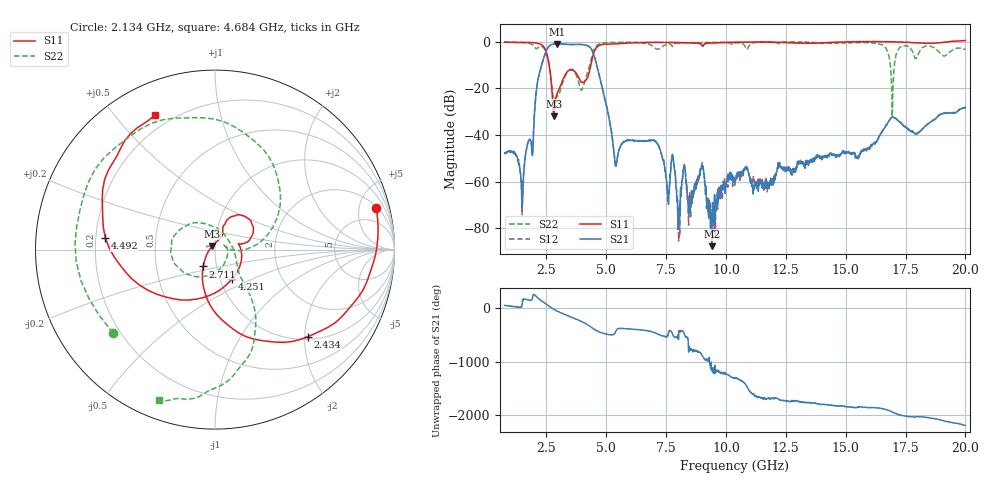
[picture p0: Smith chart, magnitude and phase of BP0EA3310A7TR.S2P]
! s2p File.  Ports: 1,3
# MHz S DB R 50
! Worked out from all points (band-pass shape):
!   1601 points, 750 MHz to 20 GHz, reference 50 ohm
!   highest |S21| = -0.91 dB at 2.94 GHz (marker M1); lowest = -87.8 dB at 9.4 GHz (marker M2)
!   |S21| within 3 dB of the highest: 2.491 GHz to 4.416 GHz (1.925 GHz wide, 55.7 % of centre)
!   lowest |S11| = -32.1 dB at 2.807 GHz (marker M3), VSWR 1.05, Z = 48.4 + j1.9 ohm
!   |S11| at or under -10 dB: 2.611 GHz to 4.348 GHz (1.737 GHz wide, 49.9 % of centre)
!   |S22| runs from -32.2 to 0.0 dB; largest |S21 - S12| = 0.0074
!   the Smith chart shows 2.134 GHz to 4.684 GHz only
!   S11 on the Smith chart (normalised r, x): 2.134 GHz: 2.21, +7.28; 2.434 GHz: 1.07, -2.08; 2.711 GHz: 0.86, -0.16; 4.251 GHz: 1.13, -0.39; 4.492 GHz: 0.24, +0.05; 4.684 GHz: 0.14, +0.64
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750  -0.15 135.7  -47.79 56.6  -47.82 56.8  -0.19 159.8
1495.94  -0.34 80.9  -67.99 133.8  -69.20 122.0  -0.33 118.8
1941.09  -0.41 38.2  -42.93 -107.4  -43.19 -106.6  -1.53 22.8
2133.59  -0.65 14.4  -16.87 -160.7  -16.87 -161.1  -2.69 -140.7
2434.38  -2.98 -43.0  -5.44 99.8  -5.46 99.4  -3.44 76.7
2711.09  -18.85 -124.8  -1.17 9.1  -1.19 8.6  -17.85 -2.7
2807.34  -32.09 128.2  -0.97 -16.9  -1.01 -17.2  -24.74 18.0
2939.69  -22.29 63.4  -0.91 -47.9  -0.94 -48.1  -23.60 13.5
3962.34  -17.45 13.3  -1.14 116.5  -1.16 116.3  -20.80 33.6
4251.09  -14.41 -60.7  -1.86 47.1  -1.85 46.9  -11.96 -49.8
4491.72  -4.24 174.1  -5.97 -28.9  -6.03 -29.3  -3.34 -79.2
4684.22  -1.71 114.2  -13.58 -76.3  -13.55 -76.8  -0.95 -110.5
5394.06  -0.89 7.1  -53.36 -67.6  -53.95 -68.5  -0.27 -165.8
6621.25  -0.36 -75.5  -42.67 -49.0  -42.51 -51.2  -0.60 152.4
7174.69  -0.23 -91.1  -44.53 -123.3  -44.43 -121.3  -3.14 11.9
7583.75  -0.26 -101.3  -66.90 -113.6  -69.11 -108.8  -1.06 -92.9
9003.44  -1.65 -173.7  -52.96 -157.5  -51.83 -153.3  -0.41 -169.1
9400.47  -0.58 168.3  -87.77 -22.3  -72.18 -50.5  -0.24 172.3
10375  -0.14 136.3  -60.22 138.7  -61.30 149.4  -0.60 147.1
13587.34  -0.63 61.0  -51.48 36.2  -51.59 32.5  -0.25 148.9
16799.69  -0.04 22.1  -34.18 -105.6  -34.20 -105.9  -5.95 23.9
20000  0.56 -79.0  -28.22 -26.3  -28.25 -26.3  -3.36 -163.1
